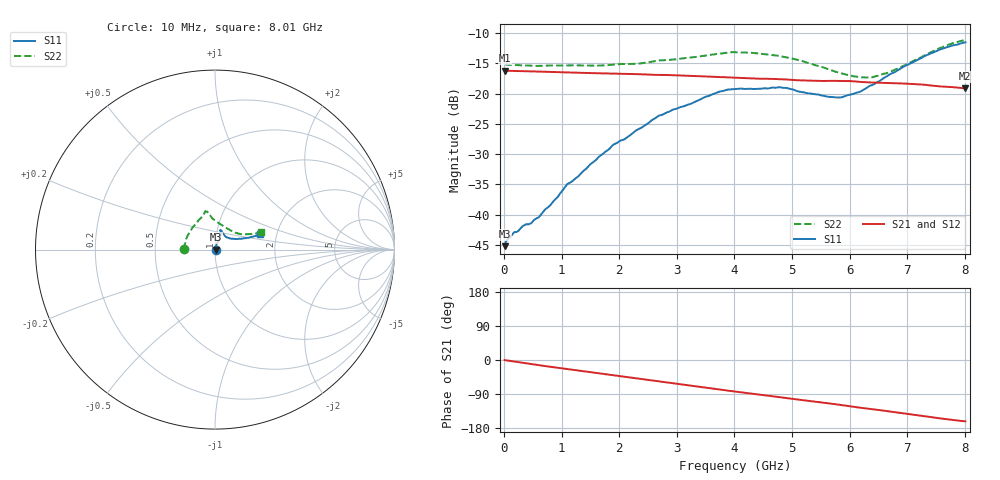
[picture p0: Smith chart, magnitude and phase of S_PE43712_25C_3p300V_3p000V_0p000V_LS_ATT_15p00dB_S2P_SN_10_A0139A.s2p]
! DEVICE ID: PE43712
! File Path: z:\PE43713\PE43713_CHAR_NOM_04292014\AMB\3p300\LS_ATT_15p00dB\PE43713_AMB_3p300V_3p000V_0p000V_LS_ATT_15p00dB_S2P_SN_10_A0139A.s2p
! Serial: 10
! Lot: A0139A
! Temp: 25C
! VDD: 3.300
! VSS: 0.000
! Control_Hi: 3.000
! Control_Lo: 0.000
! Attenuation Step: 15.00dB
! Port 1: RF1
! Port 2: RF2
! ThroughPath:1-2
! IDD: 0.0001474004
! ISS: -9.71e-008
#  Hz  S  RI  R  50
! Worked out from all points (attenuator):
!   801 points, 10 MHz to 8.01 GHz, reference 50 ohm
!   highest |S21| = -16.21 dB at 10 MHz (marker M1); lowest = -19.1 dB at 8 GHz (marker M2)
!   lowest |S11| = -45.2 dB at 10 MHz (marker M3), VSWR 1.01, Z = 50.6 + j0.0431 ohm
!   |S11| at or under -10 dB: start of sweep to end of sweep
!   |S22| runs from -17.3 to -11.2 dB; largest |S21 - S12| = 0.00055
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1e7  0.00547 0.000426  0.1548 -0.000773  0.1549 -0.000729  -0.1745 0.00117
1.6e8  0.00661 0.00236  0.154 -0.0102  0.1541 -0.0102  -0.1723 0.0119
6.1e8  0.00612 0.00738  0.1479 -0.0363  0.1479 -0.0363  -0.1651 0.0392
9.1e8  0.00519 0.0127  0.1415 -0.0521  0.1415 -0.0521  -0.1609 0.0574
1.09e9  0.0052 0.0169  0.1368 -0.0608  0.1369 -0.0608  -0.1563 0.0691
1.35e9  0.00616 0.0215  0.1298 -0.0726  0.1298 -0.0726  -0.1494 0.0833
1.9e9  0.0118 0.036  0.1115 -0.0951  0.1115 -0.0951  -0.1287 0.1172
2.11e9  0.0142 0.0401  0.1036 -0.1027  0.1036 -0.1026  -0.1213 0.1275
2.68e9  0.0257 0.0603  0.0793 -0.1189  0.0792 -0.1189  -0.0914 0.1647
3.72e9  0.0322 0.098  0.0299 -0.134  0.0298 -0.134  -0.0579 0.2057
4.01e9  0.0322 0.1046  0.0161 -0.1348  0.0161 -0.1348  -0.0546 0.2132
4.79e9  0.0326 0.1082  -0.0191 -0.1303  -0.0192 -0.1305  -0.035 0.2013
5.35e9  0.0437 0.0896  -0.0418 -0.1214  -0.0418 -0.1213  -0.0154 0.1749
5.64e9  0.0539 0.0771  -0.0524 -0.1163  -0.0524 -0.1163  0.00564 0.1585
5.87e9  0.0637 0.0685  -0.062 -0.1113  -0.0619 -0.1113  0.0259 0.1444
6.16e9  0.0815 0.0626  -0.0728 -0.102  -0.0726 -0.1021  0.0564 0.1247
6.29e9  0.0932 0.0606  -0.0762 -0.0981  -0.076 -0.0981  0.0721 0.1153
6.68e9  0.1297 0.0596  -0.0872 -0.0857  -0.087 -0.0858  0.1184 0.0927
7.37e9  0.1994 0.0703  -0.1019 -0.0583  -0.1018 -0.0583  0.1968 0.087
7.71e9  0.231 0.0787  -0.1044 -0.0451  -0.1044 -0.0452  0.2363 0.0932
8e9  0.2498 0.0888  -0.1051 -0.0343  -0.105 -0.0345  0.2572 0.0966
8.01e9  0.2504 0.0895  -0.1052 -0.0342  -0.1051 -0.0343  0.2579 0.0966
